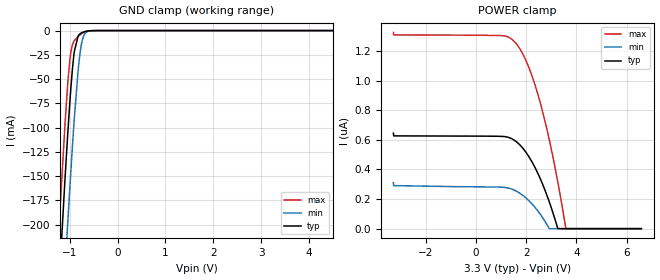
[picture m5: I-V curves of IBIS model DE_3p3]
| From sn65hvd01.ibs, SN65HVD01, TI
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|   Model
[Model]   DE_3p3
Model_type   Input
Vinl = 0.99
Vinh = 2.31
|   typ   min   max
C_comp   0.767pF   0.735pF   0.817pF
[Voltage Range]   3.3   3   3.6
[Temperature Range]   27   125   -40
[Power Clamp Reference]   3.3   3   3.6
[GND Clamp Reference]   -0   -0   -0
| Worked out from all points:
|   GND clamp passes 1 mA (typ) near -0.68 V on its own axis
[GND Clamp]
|   Voltage   I(typ)   I(min)   I(max)
-3.3V     -2.277A    -2.364A    -2.225A
-1.231V   -268.8mA   -364.6mA   -209.6mA
-1.211V   -251mA     -346.7mA   -191.9mA
-1.092V   -147.7mA   -241.5mA   -91.49mA
-1.043V   -107.7mA   -199.2mA   -55.66mA
-983.4mV  -64.12mA   -150.4mA   -24.67mA
-914.1mV  -25.42mA   -97.58mA   -11.23mA
-815.1mV  -4.94mA    -36.43mA   -5.592mA
-726mV    -1.754mA   -8.002mA   -2.426mA
-656.7mV  -721.9uA   -1.889mA   -947.7uA
-498.3mV  -42.56uA   -88.24uA   -35.49uA
6.59V     0A         0A         0A
[POWER Clamp]
|   Voltage   I(typ)   I(min)   I(max)
-3.3V     645nA      311nA      1.325uA
-3.29V    626.4nA    290.7nA    1.308uA
986.7mV   623.3nA    280.3nA    1.304uA
1.422V    606.9nA    266.9nA    1.279uA
1.67V     577.4nA    247nA      1.233uA
1.947V    524.8nA    213.4nA    1.15uA
2.224V    451.9nA    168nA      1.033uA
2.501V    358.8nA    110.4nA    884.3nA
2.927V    175.9nA    0A         593nA
3.254V    1.938nA    0A         317.8nA
3.59V     0A         0A         0A
6.59V     0A         0A         0A
